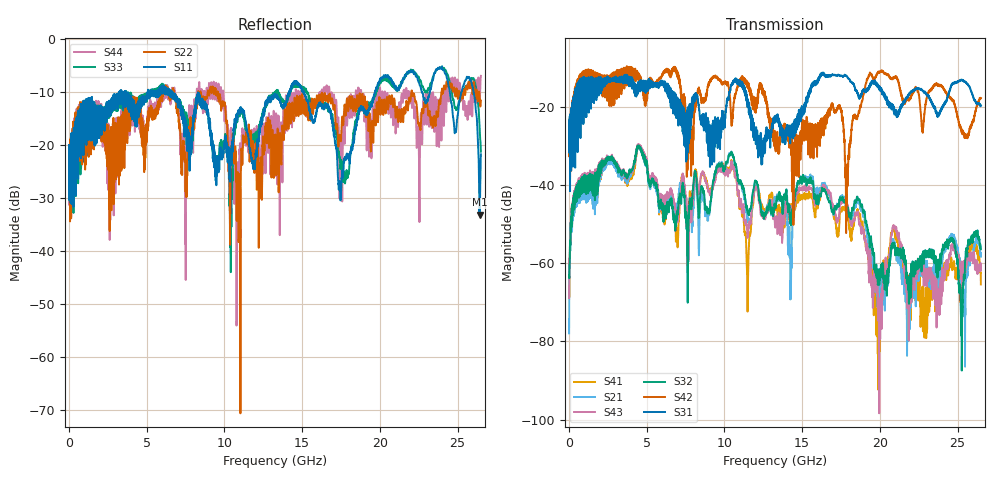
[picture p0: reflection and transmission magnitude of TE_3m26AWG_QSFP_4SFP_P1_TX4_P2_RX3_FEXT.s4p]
!Agilent Technologies,N5222A,MY51421691,A.10.00.00
!Agilent N5222A: A.10.00.00
!Date: Friday, January 30, 2015 12:38:02
!Correction: S11(Full 4 Port(1,2,3,4))
!S12(Full 4 Port(1,2,3,4))
!S13(Full 4 Port(1,2,3,4))
!S14(Full 4 Port(1,2,3,4))
!S21(Full 4 Port(1,2,3,4))
!S22(Full 4 Port(1,2,3,4))
!S23(Full 4 Port(1,2,3,4))
!S24(Full 4 Port(1,2,3,4))
!S31(Full 4 Port(1,2,3,4))
!S32(Full 4 Port(1,2,3,4))
!S33(Full 4 Port(1,2,3,4))
!S34(Full 4 Port(1,2,3,4))
!S41(Full 4 Port(1,2,3,4))
!S42(Full 4 Port(1,2,3,4))
!S43(Full 4 Port(1,2,3,4))
!S44(Full 4 Port(1,2,3,4))
!S4P File: Measurements: <S11,S12,S13,S14>,
!<S21,S22,S23,S24>,
!<S31,S32,S33,S34>,
!<S41,S42,S43,S44>:
# Hz S  dB  R 50.0
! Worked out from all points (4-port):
!   2650 points, 10 MHz to 26.5 GHz, reference 50 ohm
!   strongest paths, dB at 10 MHz, 6.63 GHz, 13.26 GHz, 19.88 GHz, 26.5 GHz:
!     S31: -24.8, -19.0, -23.3, -14.9, -19.7
!     S42: -25.1, -10.8, -28.7, -11.1, -17.7
!     S32: -63.1, -44.1, -44.8, -65.1, -56.4
!     S43: -68.9, -41.7, -49.8, -67.7, -61.8
!     S21: -77.9, -42.8, -43.2, -68.3, -58.3
!     S41: -63.7, -44.0, -45.6, -75.7, -65.4
!   lowest |S11| = -33.1 dB at 26.43 GHz (marker M1), VSWR 1.05, Z = 51.5 - j1.64 ohm
!   |S11| at or under -10 dB: start of sweep to 3.24 GHz; 6.606 GHz to 14.16 GHz (7.551 GHz wide, 72.7 % of centre); 15.11 GHz to 19.69 GHz (4.577 GHz wide, 26.3 % of centre)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
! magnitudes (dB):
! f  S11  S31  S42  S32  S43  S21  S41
! 10 MHz  -20.0  -24.8  -25.1  -63.1  -68.9  -77.9  -63.7
! 4.5 GHz  -12.5  -13.6  -12.6  -29.9  -29.6  -30.1  -30.1
! 17.87 GHz  -21.6  -12.1  -43.7  -45.5  -44.3  -44.4  -47.2
! 19.98 GHz  -8.1  -14.7  -11.3  -62.9  -72.8  -67.9  -74.0
! 20.83 GHz  -8.3  -20.4  -12.6  -55.9  -51.0  -53.8  -51.1
! 26.43 GHz  -33.1  -19.4  -17.8  -55.4  -61.3  -56.1  -59.9
! 26.5 GHz  -21.8  -19.7  -17.7  -56.4  -61.8  -58.3  -65.4
